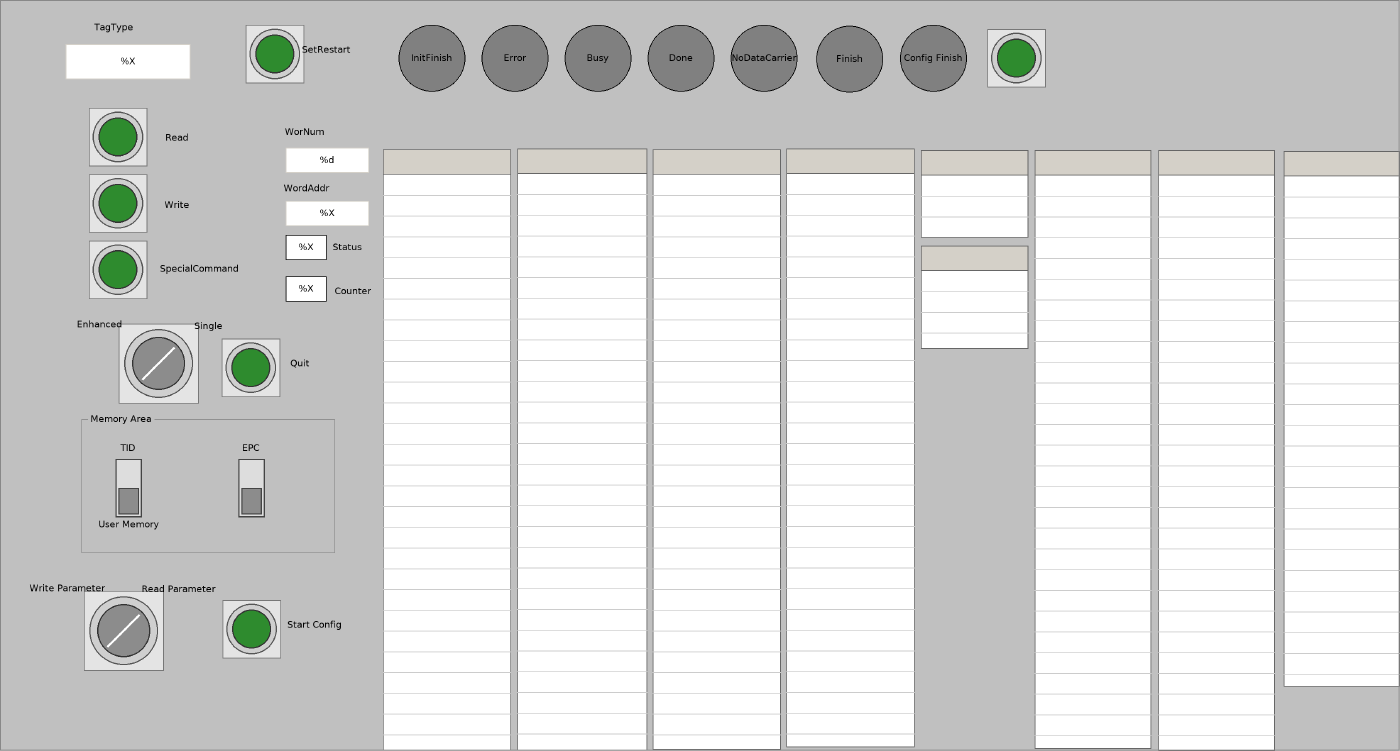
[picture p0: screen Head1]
VISUALIZATION Head1  // 1686x905
    GroupBox (98,497 305x169), "Memory Area"
        DipSwitch (22,56 70x70), variable: MAIN.Head1UserMemoryUID, behaviour: TOGGLE, style: Switch-DipSwitch-Gray
        DipSwitch (170,56 70x70), variable: MAIN.Head1EPC, behaviour: TOGGLE, style: Switch-DipSwitch-Gray
        Label (129,28 150x30), "EPC"
    PushSwitch (107,130 70x70), variable: MAIN.Head1Read, behaviour: TAP, style: Switch-PushSwitch-Green
    PushSwitch (107,210 70x70), variable: MAIN.Head1Write, behaviour: TAP, style: Switch-PushSwitch-Green
    RotarySwitch (138,390 106x96), variable: MAIN.Head1SingleEnhanced, behaviour: TOGGLE, style: Switch-RotarySwitch-Gray
    Textfield (79,53 150x42), "%X", tooltip "TagType", text variable: MAIN.Head1TagType
        OnMouseDown: write MAIN.Head1TagType via Default
    Table (461,180 154x724), data array: MAIN.IC_KP2_2HB21_IUH_MF_Head1.IDENTControl_FB_MF.INDATA
        p1892666644: MAIN.Data_Channel.InData[2][INDEX]
        p3854506369: MAIN.IC_KP2_2HB21_IUH_MF_Head1.IDENTControl_FB_MF.INDATA[INDEX]
    Table (623,179 156x725), data array: MAIN.IC_KP2_2HB21_IUH_MF_Head1.IDENTControl_FB_MF.OUTDATA
        p1892666644: MAIN.Data_Channel.OutData[2][INDEX]
        p3854506369: MAIN.IC_KP2_2HB21_IUH_MF_Head1.IDENTControl_FB_MF.OUTDATA[INDEX]
        Columns.Column.[0].Template: OnMouseDown: write the text variable via Default
    Textfield (344,242 100x30), "%X", text variable: MAIN.Head1StartAddress
        OnMouseClick: write MAIN.Head1StartAddress via Default
    Textfield (344,178 100x30), "%d", text variable: MAIN.Head1WordNum
        OnMouseClick: write MAIN.Head1WordNum via Default
    PushSwitch (296,30 70x70), variable: MAIN.Head1SetRestart, behaviour: TAP, style: Switch-PushSwitch-Green
    PushSwitch (267,408 70x70), tooltip "Cancel "Enhanced"-Command", variable: MAIN.Head1Quit, behaviour: TAP, style: Switch-PushSwitch-Green
    PushSwitch (107,290 70x70), variable: MAIN.Head1SpecialCommand, behaviour: TAP, style: Switch-PushSwitch-Green
    Table (1546,182 140x645), data array: MAIN.Head1Data.SpecialCommand
        p1892666644: MAIN.Data_Channel.SpecialCommand[2][INDEX]
        p3854506369: MAIN.Head1Data.SpecialCommand[INDEX]
        Columns.Column.[0].Template: OnMouseDown: write the text variable via Default
    Rectangle (344,283 49x30), "%X", text variable: MAIN.Head1Status, input disabled if: TRUE
    Rectangle (344,333 49x30), "%X", text variable: MAIN.Head1ReplyCounter, input disabled if: TRUE
    Ellipse (480,30 80x80), "InitFinish", colour toggle: MAIN.Head1InitFinish
    Ellipse (580,30 80x80), "Error", colour toggle: MAIN.Head1Error
    Ellipse (680,30 80x80), "Busy", colour toggle: MAIN.Head1Busy
    Ellipse (780,30 80x80), "Done", colour toggle: MAIN.Head1Done
    Ellipse (880,30 80x80), "NoDataCarrier", colour toggle: MAIN.Head1NoDataCarrier
    Label (62,18 150x30), "TagType"
    Label (292,144 150x30), "WorNum"
    Label (294,212 150x30), "WordAddr"
    Label (343,283 150x30), "Status"
    Label (350,336 150x30), "Counter"
    Label (138,151 150x30), "Read"
    Label (138,232 150x30), "Write"
    Label (165,309 150x30), "SpecialCommand"
    Label (45,376 150x30), "Enhanced"
    Label (176,378 150x30), "Single"
    Label (286,423 150x30), "Quit"
    Label (79,525 150x30), "TID"
    Label (80,617 150x30), "User Memory"
    Ellipse (983,31 80x80), "Finish", colour toggle: MAIN.Head1Finish
    Table (786,180 154x723), data array: MAIN.Head1Data.ReadData
        p1892666644: MAIN.Data_Channel.SpecialCommand[2][INDEX]
        p3854506369: MAIN.Head1Data.ReadData[INDEX]
        Columns.Column.[0].Template: OnMouseDown: write the text variable via Default
    Table (947,179 154x721), data array: MAIN.Head1Data.WriteData
        p1892666644: MAIN.Data_Channel.SpecialCommand[2][INDEX]
        p3854506369: MAIN.Head1Data.WriteData[INDEX]
        Columns.Column.[0].Template: OnMouseDown: write the text variable via Default
    Label (318,45 150x30), "SetRestart"
    RotarySwitch (96,712 106x96), variable: MAIN.Head1WriteParameter, behaviour: TOGGLE, style: Switch-RotarySwitch-Gray
    Label (140,695 150x30), "Read Parameter"
    Label (6,694 150x30), "Write Parameter"
    PushSwitch (268,723 70x70), variable: MAIN.Head1StartConfig, behaviour: TAP, style: Switch-PushSwitch-Green
    Label (304,739 150x28), "Start Config"
    Ellipse (1084,30 80x80), "Config Finish", colour toggle: MAIN.Head1EndConfig
    PushSwitch (1189,35 70x70), variable: MAIN.Head1NewData, behaviour: TAP, style: Switch-PushSwitch-Green
    Table (1109,181 129x105), data array: MAIN.Head1Data.NumberTags
        p1892666644: MAIN.Data_Channel.SpecialCommand[2][INDEX]
        p3854506369: MAIN.Head1Data.NumberTags[INDEX]
        Columns.Column.[0].Template: OnMouseDown: write the text variable via Default
    Table (1246,181 140x721), data array: MAIN.Head1Data.EPC_LeaveTag
        p1892666644: MAIN.Data_Channel.SpecialCommand[2][INDEX]
        p3854506369: MAIN.Head1Data.EPC_LeaveTag[INDEX]
        Columns.Column.[0].Template: OnMouseDown: write the text variable via Default
    Table (1395,181 140x724), data array: MAIN.Head1Data.EPC_WrittenTag
        p1892666644: MAIN.Data_Channel.SpecialCommand[2][INDEX]
        p3854506369: MAIN.Head1Data.EPC_WrittenTag[INDEX]
        Columns.Column.[0].Template: OnMouseDown: write the text variable via Default
    Table (1109,296 129x124), data array: MAIN.Head1Data.TagInformation
        p1892666644: MAIN.Data_Channel.SpecialCommand[2][INDEX]
        p3854506369: MAIN.Head1Data.TagInformation[INDEX]
        Columns.Column.[0].Template: OnMouseDown: write the text variable via Default
END_VISUALIZATION
